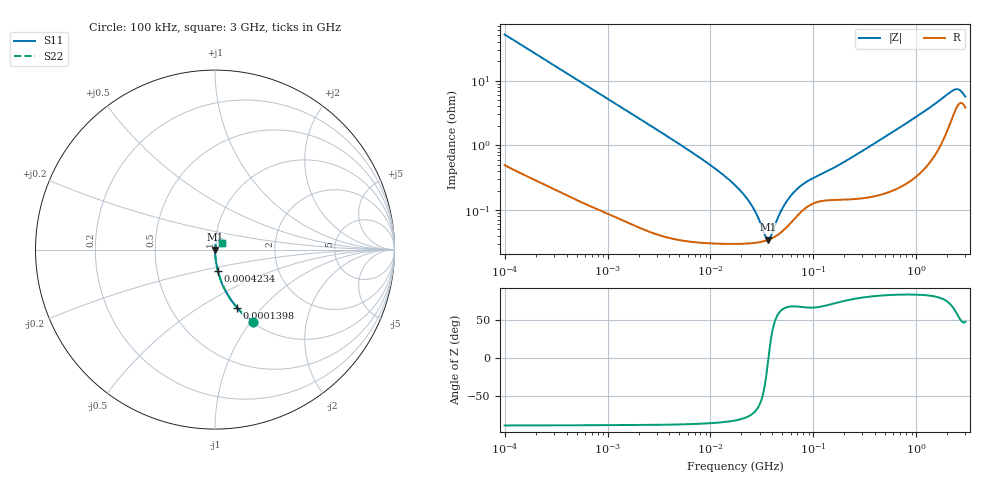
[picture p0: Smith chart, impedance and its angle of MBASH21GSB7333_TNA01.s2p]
! MBASH21GSB7333_TNA01  S-PARAMETER MODEL  ( Standard Model )
! Model Generated by TAIYO YUDEN Corporation (http://www.ty-top.com)
! Version 1.0
! TAIYO YUDEN Control No. 220601
! Copyright(c) 2013 TAIYO YUDEN CO.,LTD. All Rights Reserved.
! Product Description (link to TY-COMPAS)
! https://ds.yuden.co.jp/TYCOMPAS/or/detail?pn=MBASH21GSB7333KTNA01&u=M
! Products Name : Multilayer Ceramic Capacitors
! Characteristics :
!  Capacitance : 0.033 [uF] , Rated Voltage : 100 [V] , TCC : X7R
!  Case Size : 2.0 x 1.25 / 0.079 x 0.049 [mm/inch] , Thickness : 1.25 / 0.049 [mm/inch]
!  (Conditions: Temperature = 25 [degC] , DC Bias Voltage = 0 [V])
! External Node Assignments :
!  1  o---| |---o  2
! GND o---------o GND
! Frequency Range : 100kHz  -  3GHz  [ 401 STEP ]
# MHZ S RI R 50
! Freq[MHz].  S11 Real  S11 Imag  S21 Real  S21 Imag  S12 Real  S12 Imag  S22 Real  S22 Imag
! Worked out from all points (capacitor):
!   401 points, 100 kHz to 3 GHz, reference 50 ohm
!   read as one part in series: C = 30.8 nF near 105.3 kHz
!   lowest |Z| = 34.7 mohm at 36.57 MHz (marker M1)
!   series resonance near 36.66 MHz, so ESL is about 610 pH
!   S11 on the Smith chart (normalised r, x): 100 kHz: 1.01, -1.03; 139.8 kHz: 1.01, -0.74; 423.4 kHz: 1.00, -0.25; 3 GHz: 1.08, +0.08
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0.1  0.2127 -0.4044  0.7873 0.4044  0.7873 0.4044  0.2127 -0.4044
0.1398  0.1229 -0.3232  0.8771 0.3232  0.8771 0.3232  0.1229 -0.3232
0.228123  0.0514 -0.2151  0.9486 0.2151  0.9486 0.2151  0.0514 -0.2151
0.423445  0.0164 -0.1208  0.9836 0.1208  0.9836 0.1208  0.0164 -0.1208
0.562235  0.00982 -0.0918  0.9902 0.0918  0.9902 0.0918  0.00982 -0.0918
3.161081  0.000685 -0.0166  0.9993 0.0166  0.9993 0.0166  0.000685 -0.0166
9.574722  0.000333 -0.00518  0.9997 0.00518  0.9997 0.00518  0.000333 -0.00518
17.7727  0.000305 -0.00231  0.9997 0.00231  0.9997 0.00231  0.000305 -0.00231
25.49486  0.000309 -0.0011  0.9997 0.0011  0.9997 0.0011  0.000309 -0.0011
29.00125  0.000316 -0.000701  0.9997 0.000701  0.9997 0.000701  0.000316 -0.000701
33.85116  0.000333 -0.000238  0.9997 0.000238  0.9997 0.000238  0.000333 -0.000238
36.57227  0.000347 -6.79e-06  0.9997 6.79e-06  0.9997 6.79e-06  0.000347 -6.79e-06
39.51212  0.000366 0.000225  0.9996 -0.000225  0.9996 -0.000225  0.000366 0.000225
48.55934  0.000452 0.000857  0.9995 -0.000857  0.9995 -0.000857  0.000452 0.000857
56.67997  0.00057 0.00134  0.9994 -0.00134  0.9994 -0.00134  0.00057 0.00134
71.47675  0.00085 0.00203  0.9992 -0.00203  0.9992 -0.00203  0.00085 0.00203
97.38194  0.00125 0.00279  0.9988 -0.00279  0.9988 -0.00279  0.00125 0.00279
190.323  0.00147 0.00509  0.9985 -0.00509  0.9985 -0.00509  0.00147 0.00509
547.5153  0.00211 0.0147  0.9979 -0.0147  0.9979 -0.0147  0.00211 0.0147
2259.438  0.0308 0.0608  0.9692 -0.0608  0.9692 -0.0608  0.0308 0.0608
2570.185  0.0441 0.0544  0.9559 -0.0544  0.9559 -0.0544  0.0441 0.0544
3000  0.0384 0.0384  0.9616 -0.0384  0.9616 -0.0384  0.0384 0.0384
